FUNCTION FC 1 : VOID
BEGIN
	L		W#16#1234
	T		MW 0
	CALL		FC 2
END_FUNCTION


FUNCTION FC 2 : VOID
BEGIN
	L		W#16#6789
	T		MW 0
	L		10
	T		LB 0
END_FUNCTION


FUNCTION FC 3 : VOID
BEGIN
	L		1
	T		LB 0
	CALL		FC 2
	__ASSERT==	LB 0,	1
END_FUNCTION


ORGANIZATION_BLOCK OB 1
BEGIN
	CALL		FC 1
	__ASSERT==	MW 0,	W#16#6789
	L		0
	T		MW 0
	__ASSERT==	MW 0,	0
	UC		FC 1
	__ASSERT==	MW 0,	W#16#6789
	L		0
	T		MW 0
	__ASSERT==	MW 0,	0
	SET
	CC		FC 1
	__ASSERT==	MW 0,	W#16#6789
	L		0
	T		MW 0
	__ASSERT==	MW 0,	0
	CLR
	CC		FC 1
	__ASSERT==	MW 0,	0

	// Test localdata stack
	L		255
	T		LB 0
	__ASSERT==	LB 0,	255
	CALL		FC 3
	__ASSERT==	LB 0,	255
END_ORGANIZATION_BLOCK
